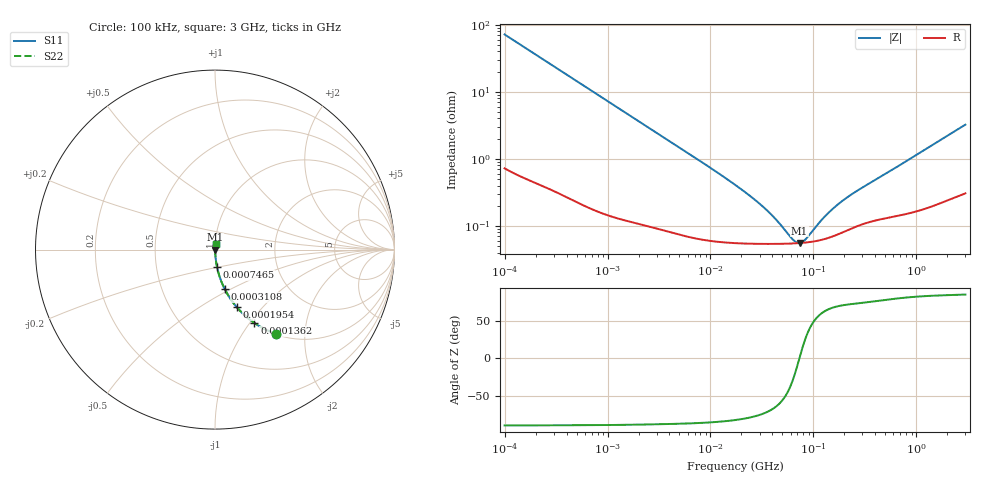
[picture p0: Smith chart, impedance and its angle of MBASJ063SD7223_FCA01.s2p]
! MBASJ063SD7223_FCA01  S-PARAMETER MODEL  ( Standard Model )
! Model Generated by TAIYO YUDEN Corporation (http://www.ty-top.com)
! Version 1.0
! TAIYO YUDEN Control No. 220601
! Copyright(c) 2022 TAIYO YUDEN CO.,LTD. All Rights Reserved.
! Product Description (link to TY-COMPAS)
! https://ds.yuden.co.jp/TYCOMPAS/or/detail?pn=MBASJ063SD7223KFCA01&u=M
! Products Name : Multilayer Ceramic Capacitors
! Characteristics :
!  Capacitance : 0.022 [uF] , Rated Voltage : 6.3 [V] , TCC : X7T
!  Case Size : 0.6 x 0.3 / 0.024 x 0.012 [mm/inch] , Thickness : 0.3 / 0.012 [mm/inch]
!  (Conditions: Temperature = 25 [degC] , DC Bias Voltage = 0 [V])
! External Node Assignments :
!  1  o---| |---o  2
! GND o---------o GND
! Frequency Range : 100kHz  -  3GHz  [ 401 STEP ]
# MHZ S RI R 50
! Freq[MHz].  S11 Real  S11 Imag  S21 Real  S21 Imag  S12 Real  S12 Imag  S22 Real  S22 Imag
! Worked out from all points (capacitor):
!   401 points, 100 kHz to 3 GHz, reference 50 ohm
!   read as one part in series: C = 22.2 nF near 105.3 kHz
!   lowest |Z| = 55.4 mohm at 73.34 MHz (marker M1)
!   series resonance near 73.22 MHz, so ESL is about 210 pH
!   S11 on the Smith chart (normalised r, x): 100 kHz: 1.01, -1.43; 136.2 kHz: 1.01, -1.05; 195.4 kHz: 1.01, -0.74; 310.8 kHz: 1.01, -0.46; 746.5 kHz: 1.00, -0.19; 3 GHz: 1.01, +0.06
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0.1  0.3407 -0.4689  0.6593 0.4689  0.6593 0.4689  0.3407 -0.4689
0.136243  0.2196 -0.4086  0.7804 0.4086  0.7804 0.4086  0.2196 -0.4086
0.19544  0.1221 -0.3215  0.8779 0.3215  0.8779 0.3215  0.1221 -0.3215
0.310802  0.0539 -0.2189  0.9461 0.2189  0.9461 0.2189  0.0539 -0.2189
0.562235  0.0183 -0.1263  0.9817 0.1263  0.9817 0.1263  0.0183 -0.1263
0.746515  0.011 -0.0961  0.989 0.0961  0.989 0.0961  0.011 -0.0961
1.421866  0.00384 -0.051  0.9962 0.051  0.9962 0.051  0.00384 -0.051
3.161081  0.00143 -0.0232  0.9986 0.0232  0.9986 0.0232  0.00143 -0.0232
9.093698  0.000674 -0.00806  0.9993 0.00806  0.9993 0.00806  0.000674 -0.00806
17.7727  0.000567 -0.00395  0.9994 0.00395  0.9994 0.00395  0.000567 -0.00395
32.98988  0.000542 -0.00181  0.9995 0.00181  0.9995 0.00181  0.000542 -0.00181
43.80277  0.00054 -0.0011  0.9995 0.0011  0.9995 0.0011  0.00054 -0.0011
62.83488  0.000547 -0.000315  0.9995 0.000315  0.9995 0.000315  0.000547 -0.000315
67.88584  0.00055 -0.000155  0.9995 0.000155  0.9995 0.000155  0.00055 -0.000155
73.34282  0.000554 3.38e-06  0.9994 -3.38e-06  0.9994 -3.38e-06  0.000554 3.38e-06
81.30716  0.000561 0.000215  0.9994 -0.000215  0.9994 -0.000215  0.000561 0.000215
97.38194  0.000581 0.000593  0.9994 -0.000593  0.9994 -0.000593  0.000581 0.000593
132.6759  0.000646 0.00129  0.9994 -0.00129  0.9994 -0.00129  0.000646 0.00129
185.4806  0.000785 0.00213  0.9992 -0.00213  0.9992 -0.00213  0.000785 0.00213
266.0711  0.000998 0.00318  0.999 -0.00318  0.999 -0.00318  0.000998 0.00318
547.5153  0.00137 0.00633  0.9986 -0.00633  0.9986 -0.00633  0.00137 0.00633
3000  0.00407 0.032  0.9959 -0.032  0.9959 -0.032  0.00407 0.032
